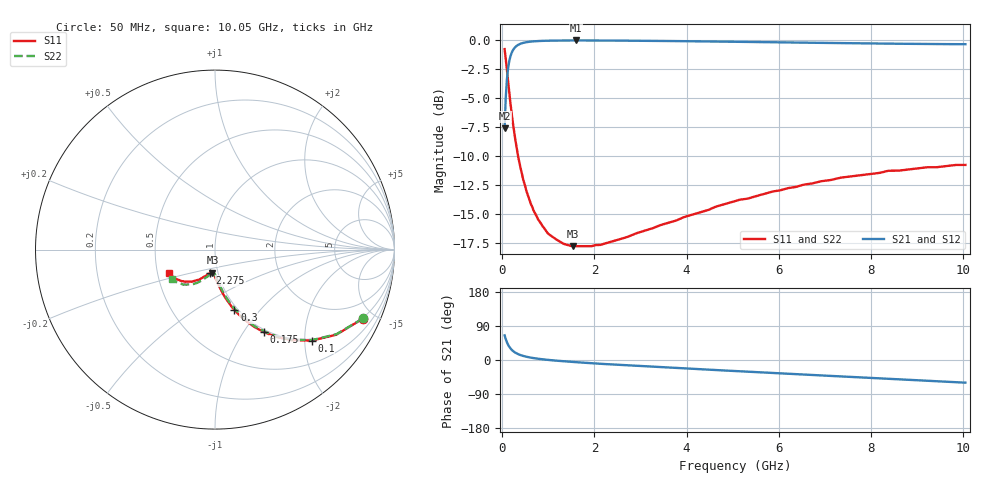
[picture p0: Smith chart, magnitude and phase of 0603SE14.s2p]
! AVX Thin Film Operation		Date: August 2001
! Description: Accu-P® Series, Thin Film, SMD, RF Capacitor
! Part Number: 06033J14FBT
! 50 MHz  -  10.05 GHz
! Serial Measurements
# mhz S db R 50
!	S11		S21		S12		S22
!	dB	Phase	dB	Phase	dB	Phase	dB	Phase
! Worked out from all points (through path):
!   401 points, 50 MHz to 10.05 GHz, reference 50 ohm
!   highest |S21| = -0.08 dB at 1.6 GHz (marker M1); lowest = -7.6 dB at 50 MHz (marker M2)
!   group delay of S21, straight-line fit = 19.9 ps
!   lowest |S11| = -17.8 dB at 1.525 GHz (marker M3), VSWR 1.30, Z = 47.1 - j12.3 ohm
!   |S11| at or under -10 dB: 340.8 MHz to end of sweep
!   |S22| runs from -17.8 to -0.8 dB; largest |S21 - S12| = 0
!   S11 on the Smith chart (normalised r, x): 50 MHz: 0.97, -4.30; 100 MHz: 0.96, -2.16; 175 MHz: 0.96, -1.24; 300 MHz: 0.96, -0.74; 2.275 GHz: 0.92, -0.24; 10.05 GHz: 0.57, -0.16
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50  -0.82 -25.0  -7.64 65.1  -7.64 65.1  -0.82 -24.9
100  -2.62 -43.3  -3.44 46.9  -3.44 46.9  -2.62 -43.0
125  -3.60 -49.8  -2.49 40.3  -2.49 40.3  -3.60 -49.5
150  -4.56 -55.1  -1.88 35.1  -1.88 35.1  -4.56 -54.7
175  -5.43 -59.3  -1.47 30.9  -1.47 30.9  -5.43 -58.8
225  -7.05 -65.7  -0.96 24.5  -0.96 24.5  -7.05 -65.1
300  -9.06 -72.2  -0.58 18.1  -0.58 18.1  -9.06 -71.4
375  -10.69 -76.5  -0.39 13.9  -0.39 13.9  -10.69 -75.4
500  -12.69 -81.3  -0.24 9.3  -0.24 9.3  -12.69 -79.9
625  -14.21 -84.5  -0.17 6.1  -0.17 6.1  -14.21 -82.9
750  -15.27 -87.1  -0.14 3.7  -0.14 3.7  -15.27 -85.1
1025  -16.81 -91.2  -0.10 -0.1  -0.10 -0.1  -16.81 -88.7
1300  -17.52 -94.2  -0.08 -3.1  -0.08 -3.1  -17.52 -91.4
1525  -17.80 -96.3  -0.08 -5.1  -0.08 -5.1  -17.80 -93.3
1600  -17.80 -96.9  -0.08 -5.7  -0.08 -5.7  -17.80 -93.9
1725  -17.80 -98.0  -0.08 -6.8  -0.08 -6.8  -17.80 -95.0
2275  -17.52 -102.0  -0.09 -11.0  -0.09 -11.0  -17.52 -98.9
3400  -16.03 -109.9  -0.12 -18.7  -0.12 -18.7  -16.03 -105.9
5050  -13.92 -121.4  -0.19 -29.2  -0.19 -29.2  -13.92 -116.4
6725  -12.39 -132.0  -0.28 -39.4  -0.28 -39.4  -12.39 -126.0
8400  -11.30 -143.1  -0.35 -49.8  -0.35 -49.8  -11.29 -136.1
10050  -10.80 -153.6  -0.40 -59.8  -0.40 -59.8  -10.80 -145.8
